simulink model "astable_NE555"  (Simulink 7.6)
settings: Solver=ode15s  StartTime=0.0  StopTime=10  RelTol=1e-3
InitFcn:
  | clc
  | delete *.mat
StopFcn:
  | close all, clc
  | load es.mat
  | plot(x(1,:),x(2,:),x(1,:),x(3,:),x(1,:),x(4,:))
  | title('Sortie du NE 555, tension aux bornes de C, tension Vce du transistor')
  | xlabel('temps')
  | grid
libraries: fl_lib x10, elec_lib x7, nesl_utility x5

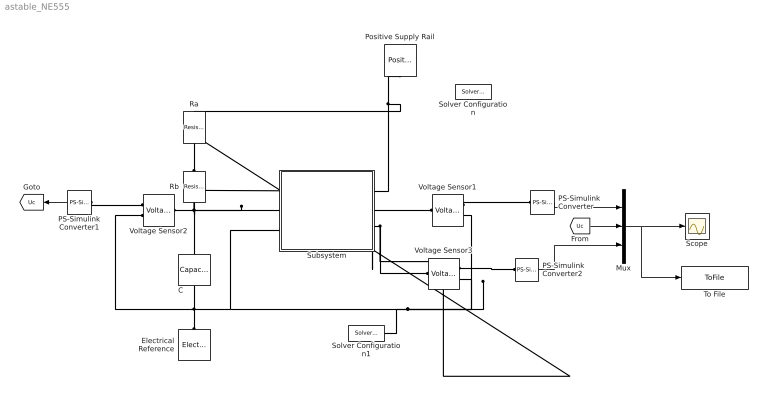
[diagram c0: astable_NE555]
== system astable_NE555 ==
  C : fl_lib/Electrical/Electrical Elements/Capacitor  DialogController=NetworkEngine.DynNeDlgSource  SystemSampleTime=-1  c=1e-3 F  v0=0 V  r=1e-6 Ohm  g=0 1/Ohm  i_Log=off  v_Log=off  vc_Log=off  LocalVarNames=|i|v|vc  LocalVarDescs=|i|v|Internal variable for voltage across capacitor term  LocalVarLogging=[0 0 0]
  Electrical Reference : fl_lib/Electrical/Electrical Elements/Electrical Reference  DialogController=NetworkEngine.DynNeDlgSource  SystemSampleTime=-1  i_Log=off  LocalVarNames=|i  LocalVarDescs=|i  LocalVarLogging=0
  Mux : Mux  Inputs=3
  PS-Simulink Converter : nesl_utility/PS-Simulink Converter  DialogController=NetworkEngine.DynNeUtilDlgSource  SystemSampleTime=-1  PhysicalDomain=network_engine_domain  LeftPortType=input  RightPortType=output  SubClassName=ps_output  Unit=1  AffineConversion=off
  PS-Simulink Converter1 : nesl_utility/PS-Simulink Converter  DialogController=NetworkEngine.DynNeUtilDlgSource  SystemSampleTime=-1  PhysicalDomain=network_engine_domain  LeftPortType=input  RightPortType=output  SubClassName=ps_output  Unit=1  AffineConversion=off
  PS-Simulink Converter2 : nesl_utility/PS-Simulink Converter  DialogController=NetworkEngine.DynNeUtilDlgSource  SystemSampleTime=-1  PhysicalDomain=network_engine_domain  LeftPortType=input  RightPortType=output  SubClassName=ps_output  Unit=1  AffineConversion=off
  Positive Supply Rail : elec_lib/Sources/Positive Supply Rail  DialogController=NetworkEngine.DynNeDlgSource  SystemSampleTime=-1  v0=5 V  current_Log=off  voltage_Log=off  power_Log=off  LocalVarNames=|current|voltage|power  LocalVarDescs=|Current (A)|Voltage (V)|Power (W)  LocalVarLogging=[0 0 0]
  Ra : fl_lib/Electrical/Electrical Elements/Resistor  DialogController=NetworkEngine.DynNeDlgSource  SystemSampleTime=-1  R=1.2 kOhm  i_Log=off  v_Log=off  LocalVarNames=|i|v  LocalVarDescs=|i|v  LocalVarLogging=[0 0]
  Rb : fl_lib/Electrical/Electrical Elements/Resistor  DialogController=NetworkEngine.DynNeDlgSource  SystemSampleTime=-1  R=1.2 kOhm  i_Log=off  v_Log=off  LocalVarNames=|i|v  LocalVarDescs=|i|v  LocalVarLogging=[0 0]
  Scope : Scope
  Solver Configuration : nesl_utility/Solver Configuration  DialogController=NetworkEngine.DynNeUtilDlgSource  SystemSampleTime=-1  PhysicalDomain=network_engine_domain  LeftPortType=input  RightPortType=generic  SubClassName=solver  Accelerate=off  Profile=off  ResidualTolerance=1e-9  MaxNonlinIter=12  MaxModeIter=2  DoFixedCost=off  UseLocalSampling=off  DoDC=off  LinearAlgebra=Sparse  LocalSolverSampleTime=.001  LocalSolverChoice=NE_BACKWARD_EULER_ADVANCER  UseLocalSolver=off
  Solver Configuration1 : nesl_utility/Solver Configuration  DialogController=NetworkEngine.DynNeUtilDlgSource  SystemSampleTime=-1  PhysicalDomain=network_engine_domain  LeftPortType=input  RightPortType=generic  SubClassName=solver  Accelerate=off  Profile=off  ResidualTolerance=1e-40  MaxNonlinIter=12  MaxModeIter=2  DoFixedCost=off  UseLocalSampling=off  DoDC=on  LinearAlgebra=Full  LocalSolverSampleTime=.001  LocalSolverChoice=NE_BACKWARD_EULER_ADVANCER  UseLocalSolver=off
  Subsystem : Subsystem
  To File : ToFile  Filename=es.mat  MatrixName=x
  Voltage Sensor1 : fl_lib/Electrical/Electrical Sensors/Voltage Sensor  DialogController=NetworkEngine.DynNeDlgSource  SystemSampleTime=-1  i1_Log=off  v1_Log=off  LocalVarNames=|i1|v1  LocalVarDescs=|i1|v1  LocalVarLogging=[]
  Voltage Sensor2 : fl_lib/Electrical/Electrical Sensors/Voltage Sensor  DialogController=NetworkEngine.DynNeDlgSource  SystemSampleTime=-1  i1_Log=off  v1_Log=off  LocalVarNames=|i1|v1  LocalVarDescs=|i1|v1  LocalVarLogging=[]
  Voltage Sensor3 : fl_lib/Electrical/Electrical Sensors/Voltage Sensor  DialogController=NetworkEngine.DynNeDlgSource  SystemSampleTime=-1  i1_Log=off  v1_Log=off  LocalVarNames=|i1|v1  LocalVarDescs=|i1|v1  LocalVarLogging=[]
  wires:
  PS-Simulink Converter1/1 -> [Uc]
  Mux/1 -> Scope/1, To File/1
  PS-Simulink Converter/1 -> Mux/1
  [Uc] -> Mux/2
  PS-Simulink Converter2/1 -> Mux/3
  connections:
  Rb/RConn1 -- Ra/LConn1 -- Subsystem/RConn3 -- Voltage Sensor3/LConn1
  Subsystem/LConn1 -- Subsystem/LConn2 -- Rb/LConn1 -- C/LConn1 -- Voltage Sensor2/LConn1
  Voltage Sensor3/RConn2 -- Voltage Sensor1/RConn2 -- C/RConn1 -- Electrical Reference/LConn1 -- Voltage Sensor2/RConn2 -- Subsystem/LConn3 -- Solver Configuration1/RConn1
  PS-Simulink Converter1/LConn1 -- Voltage Sensor2/RConn1
  Voltage Sensor1/RConn1 -- PS-Simulink Converter/LConn1
  Subsystem/RConn2 -- Voltage Sensor1/LConn1
  Voltage Sensor3/RConn1 -- PS-Simulink Converter2/LConn1
  Subsystem/RConn1 -- Positive Supply Rail/RConn1 -- Ra/RConn1

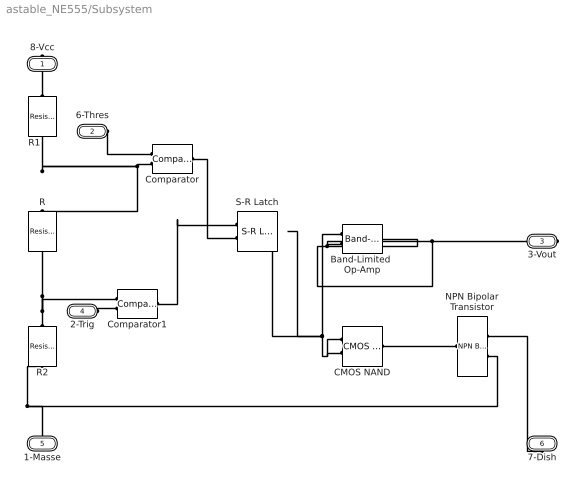
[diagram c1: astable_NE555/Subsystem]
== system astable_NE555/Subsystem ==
  Band-Limited  Op-Amp : elec_lib/Integrated Circuits/Band-Limited Op-Amp  DialogController=NetworkEngine.DynNeDlgSource  SystemSampleTime=-1  A=1000  Rin=1e+6 Ohm  Rout=100 Ohm  Vmin=-15 V  Vmax=15 V  Vdotmax=1000 V/s  f=1e+5 Hz  V0=0 V  LocalVarLogging=[]
  CMOS NAND : elec_lib/Integrated Circuits/Logic/CMOS NAND  DialogController=NetworkEngine.DynNeDlgSource  SystemSampleTime=-1  V_IL=2 V  V_IH=3 V  C_IN=5 pF  output_type=1  V_OL=0 V  V_OH=5 V  V_CC=5 V  V_meas=5 V  R_OUT=25 Ohm  R_OH=[ 25 250 ] Ohm  I_OH=63 mA  R_OL=[ 30 800 ] Ohm  I_OL=-45 mA  Delay=25 ns  Ron=5 Ohm  Vf=0.6 V  output_state=1  LocalVarLogging=[]
  Comparator : elec_lib/Integrated Circuits/Comparator  DialogController=NetworkEngine.DynNeDlgSource  SystemSampleTime=-1  V_OS=5 mV  V_OL=0 V  V_OH=5 V  C_IN=0 pF  R_OUT=50 Ohm  Delay=0 s  LocalVarLogging=[]
  Comparator1 : elec_lib/Integrated Circuits/Comparator  DialogController=NetworkEngine.DynNeDlgSource  SystemSampleTime=-1  V_OS=5 mV  V_OL=0 V  V_OH=5 V  C_IN=0 pF  R_OUT=50 Ohm  Delay=0 s  LocalVarLogging=[]
  NPN Bipolar Transistor : elec_lib/Semiconductor Devices/NPN Bipolar Transistor  DialogController=NetworkEngine.DynNeDlgSource  SystemSampleTime=-1  parameterization=1  BF=100  IS=1e-14 A  VAF=200 V  hfe=100  hoe=5e-5 1/Ohm  Ic_h=1 mA  V1=0.55 V  I1=0.5 mA  BR=1  Tmeas=25 C  RC=0.01 Ohm  RE=1e-4 Ohm  RB=1 Ohm  C_BC=5 pF  C_BE=5 pF  TF=0 us  TR=0 us  LocalVarLogging=[]
  R : fl_lib/Electrical/Electrical Elements/Resistor  DialogController=NetworkEngine.DynNeDlgSource  SystemSampleTime=-1  R=5 kOhm  i_Log=off  v_Log=off  LocalVarNames=|current|voltage|power  LocalVarDescs=|Resistor current (A)|Voltage across resistor (V)|Power (W)  LocalVarLogging=[0 0 0]
  R1 : fl_lib/Electrical/Electrical Elements/Resistor  DialogController=NetworkEngine.DynNeDlgSource  SystemSampleTime=-1  R=5 kOhm  i_Log=off  v_Log=off  LocalVarNames=|current|voltage|power  LocalVarDescs=|Resistor current (A)|Voltage across resistor (V)|Power (W)  LocalVarLogging=[0 0 0]
  R2 : fl_lib/Electrical/Electrical Elements/Resistor  DialogController=NetworkEngine.DynNeDlgSource  SystemSampleTime=-1  R=5 kOhm  i_Log=off  v_Log=off  LocalVarNames=|current|voltage|power  LocalVarDescs=|Resistor current (A)|Voltage across resistor (V)|Power (W)  LocalVarLogging=[0 0 0]
  S-R Latch : elec_lib/Integrated Circuits/Logic/S-R Latch  DialogController=NetworkEngine.DynNeDlgSource  SystemSampleTime=-1  V_IL=2 V  V_IH=3 V  C_IN=5 pF  output_type=1  V_OL=0 V  V_OH=5 V  V_CC=5 V  V_meas=5 V  R_OUT=25 Ohm  R_OH=[ 25 250 ] Ohm  I_OH=63 mA  R_OL=[ 30 800 ] Ohm  I_OL=-45 mA  Delay=25 ns  Ron=5 Ohm  Vf=0.6 V  output_state=1  LocalVarLogging=[]
  8-Vcc : PMIOPort  Port=1  Side=Right
  6-Thres : PMIOPort  Port=2  Side=Left
  3-Vout : PMIOPort  Port=3  Side=Right
  2-Trig : PMIOPort  Port=4  Side=Left
  1-Masse : PMIOPort  Port=5  Side=Left
  7-Dish : PMIOPort  Port=6  Side=Right
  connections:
  NPN Bipolar Transistor/RConn1 -- 7-Dish/RConn1
  CMOS NAND/RConn1 -- NPN Bipolar Transistor/LConn1
  NPN Bipolar Transistor/RConn2 -- R2/RConn1 -- 1-Masse/RConn1
  2-Trig/RConn1 -- Comparator1/LConn2
  6-Thres/RConn1 -- Comparator/LConn1
  8-Vcc/RConn1 -- R1/LConn1
  Comparator1/RConn1 -- S-R Latch/LConn1
  R2/LConn1 -- R/RConn1 -- Comparator1/LConn1
  Comparator/RConn1 -- S-R Latch/LConn2
  Comparator/LConn2 -- R/LConn1 -- R1/RConn1
  Band-Limited  Op-Amp/LConn2 -- Band-Limited  Op-Amp/RConn1 -- 3-Vout/RConn1
  CMOS NAND/LConn2 -- CMOS NAND/LConn1 -- Band-Limited  Op-Amp/LConn1 -- S-R Latch/RConn1
